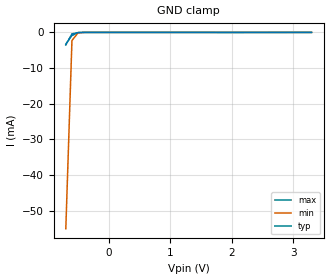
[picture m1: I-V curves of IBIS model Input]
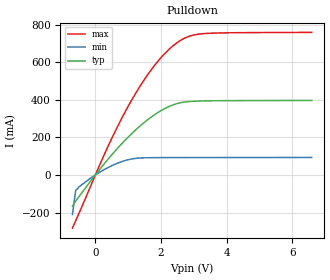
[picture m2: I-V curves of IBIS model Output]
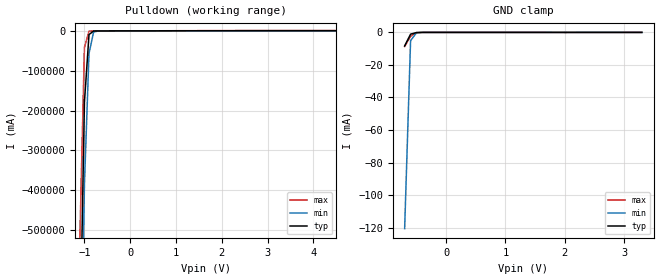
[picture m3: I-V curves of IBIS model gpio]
|IBIS model for MAX7314ATG
|created by Maxim Integrated Products
|Package model is derived for 24 pin TQFN package
[IBIS ver]   2.1
[File name]   max7314.ibs
[File Rev]   3.0
[Date]   May 27, 2009
[Source]   From Maxim Spice models.
[Notes]   IBIS 2.1 does not support differetial buffers directly;
   the I-V and V-T curves are extracted by the
   methods recommended by members of IBIS committee.
[Disclaimer]   This file is for modeling purposes only.
[Copyright]   Copyright 2009 Maxim Integrated Products.
|   Component MAX7314ATG
[Component]   MAX7314ATG
[Manufacturer]   Maxim Integrated Products
[Package]
|variable   typ   min   max
R_pkg   0.068ohm   0.059ohm   0.079ohm
L_pkg   1.132nH   0.949nH   1.319nH
C_pkg   0.107pF   0.088pF   0.128pF
[Pin] signal_name   model_name  r_pin   l_pin   c_pin
1   P0   gpio   0.079   1.318nH   0.128pF
2   P1   gpio   0.077   1.315nH   0.126pF
3   P2   gpio   0.069   1.134nH   0.109pF
4   P3   gpio   0.071   1.135nH   0.111pF
5   P4   gpio   0.077   1.315nH   0.126pF
6   P5   gpio   0.079   1.318nH   0.128pF
7   P6   gpio   0.078   1.316nH   0.127pF
8   P7   gpio   0.076   1.312nH   0.125pF
9   GND   GND   0.070   1.136nH   0.109pF
10   P8   gpio   0.071   1.137nH   0.112pF
11   P9   gpio   0.075   1.311nH   0.124pF
12   P10   gpio   0.079   1.318nH   0.128pF
13   P11   gpio   0.079   1.317nH   0.128pF
14   P12   gpio   0.077   1.315nH   0.126pF
15   P13   gpio   0.068   1.132nH   0.107pF
16   P14   gpio   0.070   1.136nH   0.111pF
17   P15   gpio   0.076   1.314nH   0.125pF
18   BLINK   Input   0.079   1.318nH   0.128pF
19   SCL   Input   0.079   1.319nH   0.126pF
20   SDA   sda   0.075   1.312nH   0.123pF
21   V+   POWER   0.069   1.133nH   0.109pF
22   INT*/O16   Output  0.067   1.130nH   0.106pF
23   RST*   Input   0.077   1.314nH   0.125pF
24   AD0   Input   0.079   1.318nH   0.128pF
| Models and submodels in the file (4): Input (Input), Output (Open_drain), gpio (I/O_open_drain), sda (I/O_open_drain)
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|   Model Input
[Model]   Input
Model_type   Input
|Signals   SCL, AD0, BLINK, RST*
Vinh = 2.3   |0.7XV+,typ
Vinl = 1.0   |0.3XV+,typ
|   typ   min   max
C_comp   2pF   1.6pF   2.5pF
[Temperature Range]   25.00   85.00   -40
[Voltage Range]   3.30V   2V   3.6V
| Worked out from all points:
|   GND clamp passes 1 mA (typ) near -0.62 V on its own axis
[GND Clamp]
|Volts   I(typ)   I(min)   I(max)
|-3.30  -2.534e+04  -2.570e+04  -2.506e+04
|-3.20  -2.383e+04  -2.420e+04  -2.354e+04
|-3.10  -2.233e+04  -2.270e+04  -2.203e+04
|-3.00  -2.083e+04  -2.121e+04  -2.052e+04
|-2.90  -1.934e+04  -1.973e+04  -1.902e+04
|-2.80  -1.786e+04  -1.826e+04  -1.752e+04
|-2.70  -1.639e+04  -1.680e+04  -1.604e+04
|-2.60  -1.494e+04  -1.535e+04  -1.457e+04
|-2.50  -1.350e+04  -1.393e+04  -1.313e+04
|-2.40  -1.211e+04  -1.254e+04  -1.173e+04
|-2.30  -1.078e+04  -1.120e+04  -1.041e+04
|-2.20  -9.577e+03  -9.944e+03  -9.282e+03
|-2.10  -8.551e+03  -8.825e+03  -8.362e+03
|-2.00  -7.668e+03  -7.865e+03  -7.516e+03
|-1.90  -6.829e+03  -7.001e+03  -6.681e+03
|-1.80  -6.002e+03  -6.171e+03  -5.849e+03
|-1.70  -5.179e+03  -5.352e+03  -5.020e+03
|-1.60  -4.362e+03  -4.541e+03  -4.196e+03
|-1.50  -3.553e+03  -3.737e+03  -3.379e+03
|-1.40  -2.754e+03  -2.946e+03  -2.571e+03
|-1.30  -1.973e+03  -2.172e+03  -1.780e+03
|-1.20  -1.224e+03  -1.429e+03  -1.021e+03
|-1.10  -5.495e+02  -7.491e+02  -3.530e+02
|-1.00  -1.006e+02  -2.297e+02  -2.160e+01
|-0.90  -4.351e+00  -2.720e+01  -2.026e-01
|-0.80  -9.694e-02  -1.368e+00  -8.379e-03
-700mV    -3.516mA   -55.04mA   -3.246mA
-600mV    -416.6uA   -2.283mA   -874uA
-500mV    -35.12uA   -99.76uA   -76.68uA
3.3V      0A         0A         0A
[POWER Clamp]
|Volts   I(typ)   I(min)   I(max)
-3.3V     0A         0A         0A
-2V       0A         0A         0A
-1V       0A         0A         0A
0V        0A         0A         0A
|   Model Output
[Model]   Output
Model_type   Open_drain
|SIGNALS   INT*/O16
|   typ   min   max
C_comp   2pF   1.6pF   2.5pF
[Temperature Range]   25.00   85.00   -40
[Voltage Range]   3.30V   2V   3.6V
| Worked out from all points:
|   slope of the pulldown table from 0 to 0.495 V, typ, clamps not added: 4.66 ohm
[PULLDOWN]
|Volts   I(typ)   I(min)   I(max)
|-3.30  -3.114e+04  -3.157e+04  -3.079e+04
|-3.20  -2.937e+04  -2.981e+04  -2.901e+04
|-3.10  -2.761e+04  -2.806e+04  -2.724e+04
|-3.00  -2.586e+04  -2.631e+04  -2.547e+04
|-2.90  -2.411e+04  -2.457e+04  -2.371e+04
|-2.80  -2.237e+04  -2.284e+04  -2.196e+04
|-2.70  -2.064e+04  -2.112e+04  -2.022e+04
|-2.60  -1.893e+04  -1.942e+04  -1.849e+04
|-2.50  -1.724e+04  -1.774e+04  -1.679e+04
|-2.40  -1.559e+04  -1.610e+04  -1.513e+04
|-2.30  -1.401e+04  -1.450e+04  -1.356e+04
|-2.20  -1.254e+04  -1.299e+04  -1.217e+04
|-2.10  -1.126e+04  -1.162e+04  -1.099e+04
|-2.00  -1.012e+04  -1.040e+04  -9.897e+03
|-1.90  -9.035e+03  -9.292e+03  -8.806e+03
|-1.80  -7.954e+03  -8.210e+03  -7.720e+03
|-1.70  -6.880e+03  -7.140e+03  -6.638e+03
|-1.60  -5.812e+03  -6.079e+03  -5.561e+03
|-1.50  -4.754e+03  -5.029e+03  -4.493e+03
|-1.40  -3.710e+03  -3.993e+03  -3.437e+03
|-1.30  -2.687e+03  -2.979e+03  -2.402e+03
|-1.20  -1.703e+03  -2.002e+03  -1.407e+03
|-1.10  -8.089e+02  -1.100e+03  -5.215e+02
|-1.00  -1.791e+02  -3.854e+02  -4.158e+01
|-0.90  -9.325e+00  -5.653e+01  -7.450e-01
|-0.80  -3.823e-01  -3.083e+00  -3.241e-01
-700mV    -165.8mA   -210.7mA   -283.2mA
-600mV    -138.7mA   -82.6mA    -244.1mA
-200mV    -45.77mA   -24.04mA   -82.46mA
300mV     65.75mA    31.35mA    119.4mA
600mV     127.1mA    57.07mA    230.7mA
900mV     183.8mA    76.22mA    333.2mA
1.4V      266.3mA    90.56mA    483mA
1.9V      331.4mA    92.1mA     603.9mA
2.4V      374.9mA    92.38mA    691.9mA
2.8V      389.7mA    92.48mA    734.2mA
3.3V      393.9mA    92.56mA    752.2mA
6.6V      396.7mA    93.19mA    758.9mA
[Ramp]
|Variable   typ   min   max
dV/dt_r  1.98/40.00n  1.18/64.00n  2.22/30.00n
dV/dt_f  1.99/400.00n  1.21/4300.00n  1.38/100.00n
R_load=4.7k
|   Model gpio
[Model]   gpio
Model_type   I/O_open_drain
|SIGNALS   P0-P15
Vinh = 2.3   |0.7XV+,typ
Vinl = 1.0   |0.3XV+,typ
|   typ   min   max
C_comp   2pF   1.6pF   2.5pF
[Temperature Range]   25.00   85.00   -40
[Voltage Range]   3.30V   2V   3.6V
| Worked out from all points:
|   slope of the pulldown table from 0 to 0.495 V, typ, clamps not added: 4.66 ohm
|   GND clamp passes 1 mA (typ) near -0.59 V on its own axis
[GND Clamp]
|Volts   I(typ)   I(min)   I(max)
|-3.30  -3.114e+04  -3.157e+04  -3.079e+04
|-3.20  -2.937e+04  -2.981e+04  -2.901e+04
|-3.10  -2.761e+04  -2.806e+04  -2.724e+04
|-3.00  -2.586e+04  -2.631e+04  -2.547e+04
|-2.90  -2.411e+04  -2.457e+04  -2.371e+04
|-2.80  -2.237e+04  -2.284e+04  -2.196e+04
|-2.70  -2.064e+04  -2.112e+04  -2.022e+04
|-2.60  -1.893e+04  -1.942e+04  -1.849e+04
|-2.50  -1.724e+04  -1.774e+04  -1.679e+04
|-2.40  -1.559e+04  -1.610e+04  -1.513e+04
|-2.30  -1.401e+04  -1.450e+04  -1.356e+04
|-2.20  -1.254e+04  -1.299e+04  -1.217e+04
|-2.10  -1.126e+04  -1.162e+04  -1.099e+04
|-2.00  -1.012e+04  -1.040e+04  -9.897e+03
|-1.90  -9.035e+03  -9.291e+03  -8.806e+03
|-1.80  -7.954e+03  -8.209e+03  -7.719e+03
|-1.70  -6.880e+03  -7.140e+03  -6.637e+03
|-1.60  -5.812e+03  -6.079e+03  -5.561e+03
|-1.50  -4.754e+03  -5.029e+03  -4.493e+03
|-1.40  -3.709e+03  -3.993e+03  -3.437e+03
|-1.30  -2.686e+03  -2.978e+03  -2.402e+03
|-1.20  -1.703e+03  -2.002e+03  -1.407e+03
|-1.10  -8.087e+02  -1.100e+03  -5.211e+02
|-1.00  -1.789e+02  -3.853e+02  -4.124e+01
|-0.90  -9.136e+00  -5.642e+01  -4.184e-01
|-0.80  -2.076e-01  -2.982e+00  -2.154e-02
-700mV    -8.33mA    -120.6mA   -8.654mA
-600mV    -1.082mA   -5.057mA   -2.323mA
-500mV    -91.63uA   -224.1uA   -202.8uA
3.3V      0A         0A         0A
[PULLDOWN]
|Volts   I(typ)   I(min)   I(max)
-3.3V     -31.14kA   -31.57kA   -30.79kA
-1.1V     -808.9A    -1.1kA     -521.5A
-1V       -179.1A    -385.4A    -41.58A
-900mV    -9.325A    -56.53A    -745mA
-800mV    -382.3mA   -3.083A    -324.1mA
-700mV    -165.8mA   -210.7mA   -283.2mA
6.6V      396.7mA    93.19mA    758.9mA
[Ramp]
|Variable   typ   min   max
dV/dt_r  1.98/40.00n  1.18/64.00n  2.22/30.00n
dV/dt_f  1.99/400.00n  1.21/4300.00n  1.38/100.00n
R_load=4.7k
